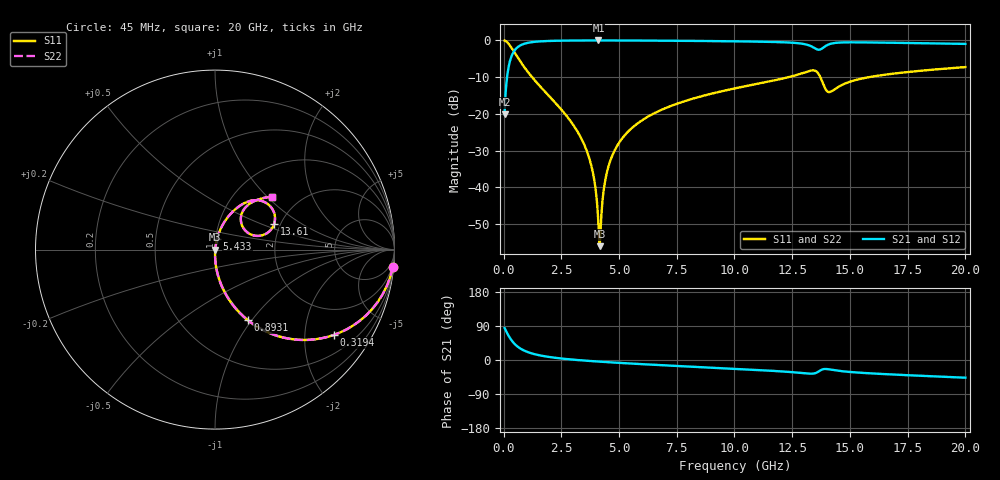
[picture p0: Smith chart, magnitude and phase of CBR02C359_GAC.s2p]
! S-parameter model data by Modelithics Inc.  support@modelithics.com 813-866-6335  Tampa FL USA
! S-Parameter data specifications:
! Substrate: 20-mil Rogers 4350B, substrate thickness, H=0.508mm, Dielectric constant, Er=3.75
! PCB Mounting Pad Footprint: Pad width, PadW=0.32mm , Pad length, PadL=0.37mm , Pad gap, PadG (edge-to-edge)=0.19mm , Reference planes=0.93mm apart
#  GHz  S  MA  R 50
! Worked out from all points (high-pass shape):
!   801 points, 45 MHz to 20 GHz, reference 50 ohm
!   highest |S21| = -0.01 dB at 4.111 GHz (marker M1); lowest = -20.1 dB at 45 MHz (marker M2)
!   |S21| within 3 dB of the highest: 446.7 MHz to end of sweep
!   lowest |S11| = -56.0 dB at 4.161 GHz (marker M3), VSWR 1.00, Z = 50.2 - j0.0102 ohm
!   |S11| at or under -10 dB: 1.235 GHz to 12.34 GHz (11.1 GHz wide, 164 % of centre); 13.72 GHz to 15.82 GHz (2.103 GHz wide, 14.2 % of centre)
!   |S22| runs from -56.0 to 0.0 dB; largest |S21 - S12| = 0
!   S11 on the Smith chart (normalised r, x): 45 MHz: 1, -20; 319.4 MHz: 0.99, -2.79; 893.1 MHz: 0.99, -0.96; 5.433 GHz: 1.02, +0.12; 13.61 GHz: 1.85, +0.62; 20 GHz: 1.47, +1.07
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0.045  0.9951 -5.7  0.09913 84.3  0.09913 84.3  0.9951 -5.7
0.194662  0.9179 -23.6  0.3964 66.4  0.3964 66.4  0.9179 -23.6
0.319381  0.8147 -35.7  0.5794 54.2  0.5794 54.2  0.8147 -35.7
0.593762  0.5973 -53.9  0.8012 36.1  0.8012 36.1  0.5973 -53.9
0.893088  0.4343 -65.1  0.8998 24.8  0.8998 24.8  0.4343 -65.1
1.691288  0.2176 -78.9  0.9748 10.8  0.9748 10.8  0.2176 -78.9
3.387462  0.04507 -89.1  0.9974 -1.0  0.9974 -1.0  0.04507 -89.1
3.861394  0.01635 -87.7  0.9982 -3.1  0.9982 -3.1  0.01635 -87.7
3.986112  0.00947 -84.1  0.9983 -3.6  0.9983 -3.6  0.00947 -84.1
4.110831  0.003058 -62.9  0.9983 -4.2  0.9983 -4.2  0.003058 -62.9
4.160719  0.001593 -3.6  0.9983 -4.4  0.9983 -4.4  0.001593 -3.6
4.23555  0.004228 63.1  0.9983 -4.7  0.9983 -4.7  0.004228 63.1
4.385212  0.01162 76.7  0.9982 -5.3  0.9982 -5.3  0.01162 76.7
4.584763  0.02133 79.6  0.998 -6.0  0.998 -6.0  0.02133 79.6
5.43285  0.05918 79.2  0.9964 -9.1  0.9964 -9.1  0.05918 79.2
6.704981  0.1089 75.7  0.992 -13.3  0.992 -13.3  0.1089 75.7
10.0225  0.2229 65.9  0.9718 -23.4  0.9718 -23.4  0.2229 65.9
13.36496  0.3911 38.2  0.8201 -36.1  0.8201 -36.1  0.3911 38.2
13.6144  0.3604 23.7  0.749 -31.5  0.749 -31.5  0.3604 23.7
14.11327  0.1984 36.7  0.8897 -24.8  0.8897 -24.8  0.1984 36.7
16.68248  0.347 51.1  0.9305 -37.8  0.9305 -37.8  0.347 51.1
20  0.4337 42.7  0.8964 -46.7  0.8964 -46.7  0.4337 42.7
